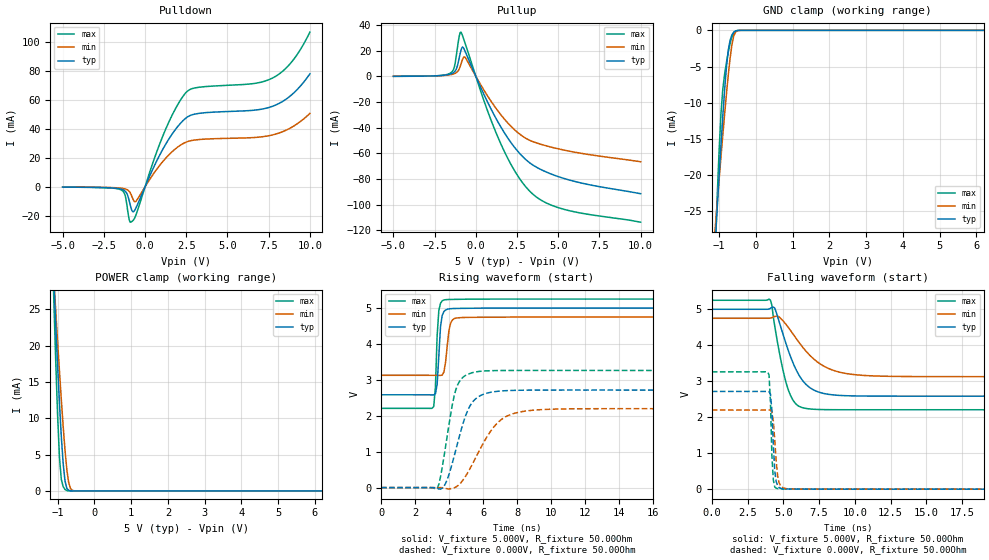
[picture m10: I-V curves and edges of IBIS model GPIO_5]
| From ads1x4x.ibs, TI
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|   GPIO 5.0V Model
[Model]   GPIO_5
Model_type   I/O
|Signals   REFP0_GPIO0 REFN0_GPIO1 AIN4_IEXC_GPIO4 AIN5_IEXC_GPIO5
|AIN6_IEXC_GPIO6 AIN7_IEXC_GPIO7 AIN2_IEXC_GPIO2 AIN3_IEXC_GPIO3
Vinl =  0.75V
Vinh =  2.00V
| variable   typ   min   max
|C_comp Output Disabled
C_comp   1.645pF   1.982pF   1.444pF
|C_comp Output Low
|C_comp   3.869pF   4.421pF   3.662pF
|C_comp Output High
|C_comp   7.463pF   6.005pF   11.333pF
[Model Spec]
|Timing spec test load voltage corners 0.5*VCC
Vmeas   2.5V   2.375V   2.625V
Vref   2.5V   2.375V   2.625V
|Junction Temperature
[Temperature Range]   40.0   105.0   -40.0
[Voltage range]   5.0V   4.75V   5.25V
[pullup reference]   5.0V   4.75V   5.25V
[power clamp reference]   5.0V   4.75V   5.25V
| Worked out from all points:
|   slope of the pulldown table from 0 to 0.75 V, typ, clamps not added: 39.9 ohm
|   slope of the pullup table from 0 to 0.75 V, typ, clamps not added: 35.6 ohm
|   GND clamp passes 1 mA (typ) near -0.68 V on its own axis
|   POWER clamp passes 1 mA (typ) near -0.78 V on its own axis
|   falling waveform, V_fixture 5.000V, R_fixture 50.00Ohm: 20-80 % time 1.44ns typ, 2.21ns min, 942ps max; typ from 5 V to 2.58 V
|   rising waveform, V_fixture 5.000V, R_fixture 50.00Ohm: 20-80 % time 185ps typ, 236ps min, 158ps max; typ from 2.58 V to 5 V
|   rising waveform, V_fixture 0.000V, R_fixture 50.00Ohm: 20-80 % time 1.01ns typ, 1.64ns min, 702ps max; typ from 0 V to 2.71 V
|   falling waveform, V_fixture 0.000V, R_fixture 50.00Ohm: 20-80 % time 193ps typ, 258ps min, 169ps max; typ from 2.71 V to 0 V
[Pulldown]
|   Voltage   I(typ)   I(min)   I(max)
-5V       -197.5uA   -151.9uA   -197.4uA
-1.45V    -1.587mA   -944.3uA   -2.142mA
-1.2V     -3.062mA   -1.489mA   -6.233mA
-950mV    -10.17mA   -3.269mA   -23.22mA
-850mV    -14.6mA    -5.228mA   -24.32mA
-700mV    -17.15mA   -9.273mA   -22.8mA
-550mV    -14.46mA   -9.917mA   -19.29mA
1.1V      26.36mA    17.76mA    35.65mA
2.45V     47.19mA    30.64mA    64.61mA
7.7V      55.42mA    35.72mA    74.85mA
8.9V      63.52mA    41.11mA    86.22mA
10V       77.92mA    50.63mA    106.7mA
[GND Clamp]
|   Voltage   I(typ)   I(min)   I(max)
-5V       -403.6mA   -288.5mA   -636.5mA
-1.1V     -28.82mA   -26.84mA   -29.34mA
-1.05V    -24.39mA   -23.68mA   -22.68mA
-1V       -20.05mA   -20.56mA   -16.59mA
-950mV    -15.85mA   -17.49mA   -11.52mA
-900mV    -11.85mA   -14.48mA   -8.111mA
-800mV    -5.026mA   -8.749mA   -4.411mA
-750mV    -2.711mA   -6.126mA   -2.987mA
-650mV    -613.9uA   -1.925mA   -868.3uA
-600mV    -244.8uA   -736.3uA   -329.6uA
-550mV    -83.37uA   -214.1uA   -95.6uA
10V       0A         0A         0A
[Pullup]
|   Voltage   I(typ)   I(min)   I(max)
-5V       -21.79uA   -10.2uA    -34.94uA
-1.55V    1.71mA     1.198mA    2.4mA
-1.3V     3.43mA     2.03mA     7.281mA
-1V       14.72mA    5.889mA    31.52mA
-900mV    20.25mA    9.482mA    34.45mA
-800mV    22.81mA    13.34mA    31.42mA
-650mV    19.44mA    14.77mA    25.73mA
1.35V     -35.75mA   -27.15mA   -47.75mA
2.35V     -55.4mA    -41.69mA   -73.58mA
3.25V     -67.27mA   -49.8mA    -89.29mA
5.35V     -79.67mA   -57.54mA   -103.7mA
10V       -91.55mA   -66.64mA   -113.8mA
[POWER Clamp]
|   Voltage   I(typ)   I(min)   I(max)
-5V       295mA      258.1mA    348.7mA
-1.15V    35.1mA     33.46mA    34.21mA
-1.1V     28.8mA     28.98mA    25.73mA
-1.05V    22.77mA    24.68mA    17.65mA
-1V       17.16mA    20.52mA    10.34mA
-950mV    12.05mA    16.49mA    4.629mA
-900mV    7.527mA    12.61mA    1.596mA
-850mV    3.818mA    8.952mA    598.3uA
-750mV    368.4uA    2.966mA    48.18uA
-650mV    17.55uA    344.3uA    1.801uA
-500mV    207nA      4.555uA    9.295nA
10V       0A         0A         0A
[Ramp]
R_load = 50.00Ohm
|   typ   min   max
dV/dt_r   1.629V/1.013ns   1.319V/1.636ns   1.957V/701.615ps
dV/dt_f   1.449V/1.444ns   973.376mV/2.214ns   1.826V/942.160ps
[Falling Waveform]
V_fixture = 5.000V
V_fixture_min = 4.750V
V_fixture_max = 5.250V
R_fixture = 50.00Ohm
|   Time   V(typ)   V(min)   V(max)
0s        5V         4.75V      5.25V
4.1ns     5.026V     4.754V     5.254V
4.4ns     5.033V     4.8V       4.528V
4.8ns     4.535V     4.751V     3.639V
5.2ns     4.027V     4.573V     2.947V
5.7ns     3.487V     4.3V       2.459V
6.3ns     3.044V     3.972V     2.269V
7.9ns     2.653V     3.404V     2.211V
9.9ns     2.592V     3.186V     2.207V
25ns      2.585V     3.128V     2.207V
[Rising Waveform]
V_fixture = 5.000V
V_fixture_min = 4.750V
V_fixture_max = 5.250V
R_fixture = 50.00Ohm
|   Time   V(typ)   V(min)   V(max)
0s        2.585V     3.128V     2.207V
3.1ns     2.582V     3.127V     2.258V
3.2ns     2.613V     3.127V     2.795V
3.3ns     2.868V     3.126V     4.221V
3.4ns     3.66V      3.125V     4.928V
3.5ns     4.486V     3.124V     5.133V
3.7ns     4.904V     3.221V     5.225V
4ns       4.977V     4.389V     5.238V
4.4ns     4.988V     4.72V      5.242V
25ns      5V         4.75V      5.25V
[Rising Waveform]
V_fixture = 0.000V
V_fixture_min = 0.000V
V_fixture_max = 0.000V
R_fixture = 50.00Ohm
|   Time   V(typ)   V(min)   V(max)
0s        2.054nV    2.521nV    1.817nV
3.3ns     -20.34mV   115.7uV    -36.07mV
3.5ns     -42.98mV   422.9uV    300.4mV
3.8ns     119.1mV    -21.62mV   1.152V
4.4ns     1.051V     15.85mV    2.727V
5ns       2.032V     336.7mV    3.132V
5.4ns     2.392V     677mV      3.204V
6.8ns     2.679V     1.777V     3.259V
8.4ns     2.712V     2.124V     3.262V
25ns      2.715V     2.198V     3.261V
[Falling Waveform]
V_fixture = 0.000V
V_fixture_min = 0.000V
V_fixture_max = 0.000V
R_fixture = 50.00Ohm
|   Time   V(typ)   V(min)   V(max)
0s        2.715V     2.198V     3.261V
3.9ns     2.718V     2.2V       3.259V
4ns       2.711V     2.201V     3.177V
4.1ns     2.642V     2.195V     2.401V
4.2ns     2.191V     2.145V     939.4mV
4.3ns     1.235V     1.898V     251.1mV
4.5ns     213mV      774.2mV    25.94mV
4.7ns     46.04mV    182.8mV    8.889mV
5.3ns     4.944mV    10.5mV     3.062mV
25ns      2.054nV    2.521nV    1.817nV
